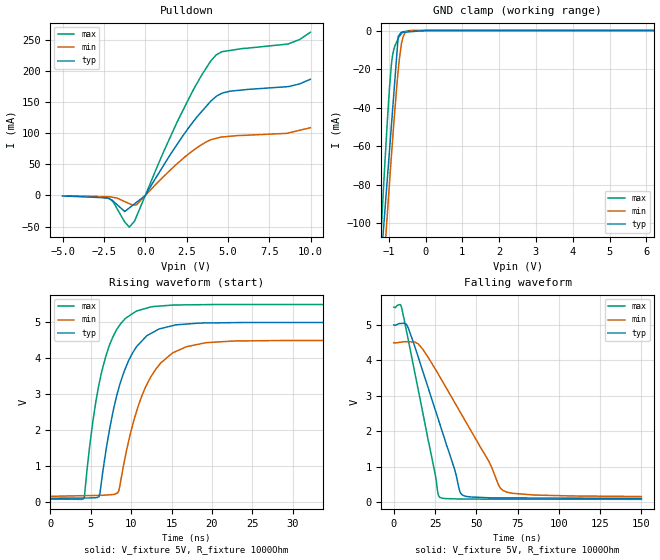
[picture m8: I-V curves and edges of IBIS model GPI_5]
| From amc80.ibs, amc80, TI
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[Model]  GPI_5
Model_type   I/O_open_drain
Polarity   Non-Inverting
Enable   Active-Low
Vinl = 0.8
Vinh = 2
Vmeas = 2.5
Vref = 2.5
Cref = 15pF
Rref = 50
|   typ   min   max
|   (nom PVT)   (Fast PVT)   (slow PVT)
|   BUFFER OUTPUT TURNED HIGH or as an INPUT
|C_comp   9.122E-13   8.552E-13   9.122E-13
|   BUFFER OUTPUT TURNED LOW
C_comp   8.552E-13   8.435E-13   9.122E-13
| Where   nom PVT is  Nominal Process, 5.0V, 27C
|   Fast PVT is Strong Process, 5.5V, -40C
|   Slow PVT is Weak Process, 4.5V, 125C
|C_comp - from L-C Tank method, L = 1nH, peak frequency
[Voltage Range]   5   4.5   5.5
[Temperature Range]   27   125   -40
[Pullup Reference]   5   4.5   5.5
[Pulldown Reference]   0   0   0
[Power Clamp Reference]   5   4.5   5.5
[GND Clamp Reference]   0   0   0
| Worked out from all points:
|   slope of the pulldown table from 0 to 0.75 V, typ, clamps not added: 22.8 ohm
|   GND clamp passes 1 mA (typ) near -0.67 V on its own axis
|   falling waveform, V_fixture 5V, R_fixture 1000Ohm: 20-80 % time 20.4ns typ, 32.1ns min, 14ns max; typ from 5 V to 0.109 V
|   rising waveform, V_fixture 5V, R_fixture 1000Ohm: 20-80 % time 3.22ns typ, 3.79ns min, 2.73ns max; typ from 0.109 V to 5 V
[Pulldown]
|   Voltage   I(typ)   I(min)   I(max)
-5V       -736.2uA   -519.2uA   -724.3uA
-2.168V   -5.497mA   -2.139mA   -4.9mA
-1.245V   -25.76mA   -9.864mA   -42.6mA
-961.1mV  -19.88mA   -13.14mA   -50.82mA
-534.5mV  -11.06mA   -14.87mA   -33.94mA
135.4uV   6.145uA    3.86uA     8.58uA
1.966V    83.48mA    51.89mA    120mA
3.435V    135.3mA    81.91mA    194mA
4.28V     158.6mA    91.6mA     225.2mA
5.124V    167.2mA    94.92mA    232.5mA
8.629V    174.5mA    99.99mA    242.9mA
9.985V    186.3mA    108.6mA    261.6mA
[GND Clamp]
|   Voltage   I(typ)   I(min)   I(max)
-5V       -1.389A    -1.299A    -1.55A
-1.232V   -125.6mA   -150.3mA   -113.6mA
-1.13V    -99.95mA   -121.1mA   -77.52mA
-1.09V    -89.91mA   -109.6mA   -64.16mA
-1.046V   -79.09mA   -97.64mA   -49.74mA
-918.8mV  -47.2mA    -62.99mA   -16.29mA
-844.3mV  -28.6mA    -43.98mA   -8.638mA
-742.3mV  -3.11mA    -20.79mA   -4.075mA
-666mV    -995.8uA   -8.462mA   -1.868mA
-549.2mV  -821.1uA   -986.9uA   -464.3uA
-346.3mV  -517.8uA   -5.329uA   -2.814uA
9.985V    0A         0A         0A
[POWER Clamp]
|   SCR cell for ESD function. Effects occurr above VDD x 2
|   Voltage   I(typ)   I(min)   I(max)
-5V       0A         0A         0A
0V        0A         0A         0A
10V       0A         0A         0A
[Ramp]
R_load = 1000
|   typ   min   max
dV/dt_r   2.93461/3.22e-009   2.6024/3.77671e-009   3.25031/2.72908e-009
dV/dt_f   2.93461/2.04117e-008   2.60233/3.21469e-008   3.25031/1.3963e-008
[Falling Waveform]
V_fixture = 5V
V_fixture_min = 4.5V
V_fixture_max = 5.5V
R_fixture = 1000Ohm
C_fixture = 0F
|   Time   V(typ)   V(min)   V(max)
0s        5V         4.5V       5.5V
4.814ns   5.043V     4.518V     5.479V
8.798ns   4.913V     4.525V     4.58V
14.75ns   4.106V     4.468V     3.19V
25.15ns   2.605V     3.756V     780.4mV
26.84ns   2.362V     3.626V     235.9mV
27.85ns   2.217V     3.544V     142.2mV
40.59ns   250mV      2.516V     91.65mV
66.21ns   123.1mV    333mV      87.96mV
150ns     109mV      162.8mV    82.82mV
[Rising Waveform]
V_fixture = 5V
V_fixture_min = 4.5V
V_fixture_max = 5.5V
R_fixture = 1000Ohm
C_fixture = 0F
|   Time   V(typ)   V(min)   V(max)
0s        109mV      162.7mV    82.82mV
4.169ns   115.2mV    180.6mV    108.1mV
6.035ns   156.6mV    188.7mV    3.291V
7.358ns   2.06V      205.9mV    4.39V
8.637ns   3.307V     494.8mV    4.944V
10.36ns   4.217V     2.298V     5.274V
12.46ns   4.696V     3.495V     5.433V
16.85ns   4.956V     4.326V     5.49V
22.69ns   4.995V     4.484V     5.499V
150ns     5V         4.5V       5.5V
